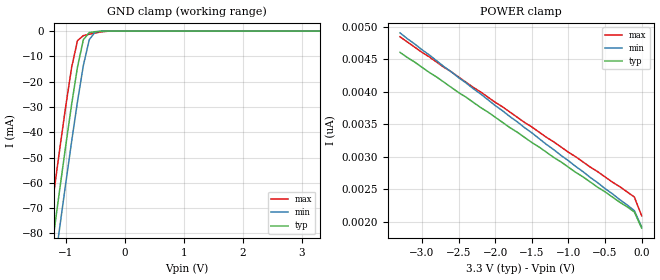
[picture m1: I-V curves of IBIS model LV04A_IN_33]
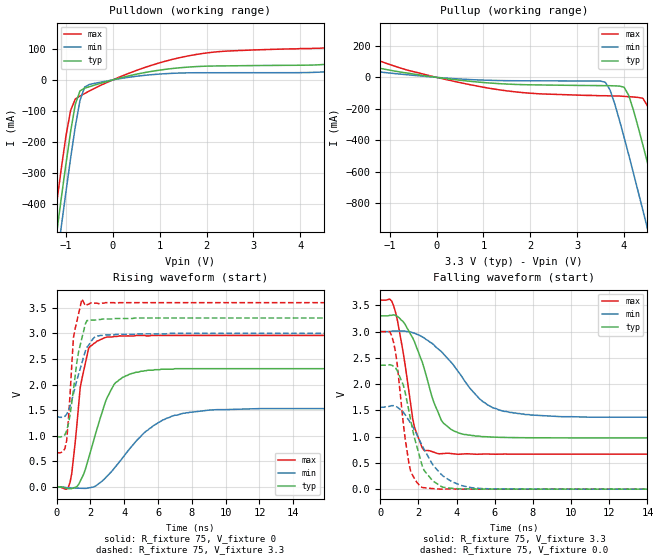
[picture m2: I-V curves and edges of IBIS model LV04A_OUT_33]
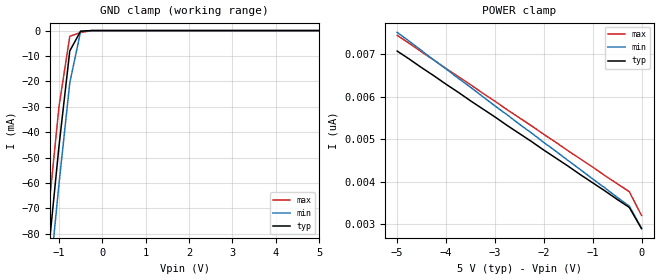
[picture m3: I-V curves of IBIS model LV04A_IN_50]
| TEXAS INSTRUMENTS INCORPORATED
| Standard Linear and Logic Group
| IBIS Model of SN74LV04A
| HEX INVERTER
| SOIC 14-pin (D), SOP 14-pin (NS), SSOP 14-pin (DB), TSSOP 14-pin (PW)
| and TVSOP 14-pin (DGV) Package
[IBIS Ver]   3.2
[Comment Char]  |_char
[File Name]   lv04a.ibs
[File Rev]   2.0 H_die
[Date]   May 26, 2000
[Source]   Data created from HSPICE simulations at TI-SLL.
[Notes]   The following is an IBIS list for the LV04A.
|   Please contact sllibis@ti.com with questions and
|   comments concerning SLL IBIS models.
|   The warning about AC Rising Endpoint might be reported,
|   but it is due to HSPICE issue and negligible.
[Disclaimer] Property of Texas Instruments Incorporated.  Unauthorized
   reproduction and/or distribution is strictly prohibited.
   This product is protected under copyright law.
   Created 2000, (C) Copyright 2000, Texas Instruments Inc.,
   All Rights Reserved.
   UNLESS THERE IS A SIGNED, WRITTEN AGREEMENT TO THE
   CONTRARY, TEXAS INSTRUMENTS () IS PROVIDING THE IBIS
   MODELS  AND WITHOUT ANY WARRANTY, EXPRESSED OR
   IMPLIED.  TI assumes no liability for:
   1) the accuracy of the IBIS models provided to your
   company;
   2) the proper functioning of these IBIS Models in your
   design or for any resulting applications; or
   3) infringement of patents, copyrights or intellectual
   property rights resulting from your use of these IBIS
   models.
   TI provides IBIS Models as a service to our customers.
   You and your company shall not distribute, sell or give
   these models to anyone else without prior written
   permission from TI.
   TI reserves the right to make changes to our products or
   to discontinue any semiconductor product or service
   without notice, and advises our customers to obtain the
   latest version of relevant information to verify, before
   placing orders, that the information being relied on is
   current.
   Please be aware that your receipt and use of the IBIS
   information provided shall serve as acceptance of these
   terms and conditions.  If you do not accept these terms,
   you should return or destroy the IBIS models and any
   other accompanying information immediately.
|   Component LV04A_D
[Component]   LV04A_D
[Manufacturer]  Texas Instruments, Inc.
[Package]
|   typ   min   max
R_pkg   0.031   0.028   0.034
L_pkg   3.109nH   2.462nH   3.889nH
C_pkg   0.473pF   0.363pF   0.628pF
[Pin]   signal_name   model_name   R_pin   L_pin   C_pin
1   1A   LV04A_IN   0.033   3.854nH   0.622pF
2   1Y   LV04A_OUT   0.032   3.188nH   0.473pF
3   2A   LV04A_IN   0.028   2.462nH   0.377pF
4   2Y   LV04A_OUT   0.031   2.596nH   0.363pF
5   3A   LV04A_IN   0.028   2.521nH   0.372pF
6   3Y   LV04A_OUT   0.034   3.250nH   0.476pF
7   GND   GND   0.034   3.889nH   0.628pF
8   4Y   LV04A_OUT   0.034   3.889nH   0.628pF
9   4A   LV04A_IN   0.034   3.250nH   0.476pF
10   5Y   LV04A_OUT   0.028   2.521nH   0.372pF
11   5A   LV04A_IN   0.031   2.596nH   0.364pF
12   6Y   LV04A_OUT   0.028   2.462nH   0.377pF
13   6A   LV04A_IN   0.032   3.188nH   0.473pF
14   VCC   POWER   0.033   3.854nH   0.622pF
|   Component LV04A_NS
[Component]   LV04A_NS
[Manufacturer]  Texas Instruments, Inc
[Package]
|   typ   min   max
R_pkg   0.045   0.039   0.054
L_pkg   3.796nH   2.561nH   4.952nH
C_pkg   0.528pF   0.288pF   0.710pF
[Pin]   signal_name   model_name   R_pin   L_pin   C_pin
1   1A   LV04A_IN   0.047   4.867nH   0.706pF
2   1Y   LV04A_OUT   0.051   4.083nH   0.592pF
3   2A   LV04A_IN   0.041   2.915nH   0.376pF
4   2Y   LV04A_OUT   0.039   2.561nH   0.288pF
5   3A   LV04A_IN   0.041   3.101nH   0.430pF
6   3Y   LV04A_OUT   0.047   4.047nH   0.589pF
7   GND   GND   0.051   4.909nH   0.700pF
8   4Y   LV04A_OUT   0.045   4.784nH   0.694pF
9   4A   LV04A_IN   0.054   4.176nH   0.597pF
10   5Y   LV04A_OUT   0.039   3.287nH   0.449pF
11   5A   LV04A_IN   0.039   2.586nH   0.294pF
12   6Y   LV04A_OUT   0.040   2.802nH   0.371pF
13   6A   LV04A_IN   0.049   4.080nH   0.593pF
14   VCC   POWER   0.052   4.952nH   0.710pF
|   Component LV04A_DB
[Component]   LV04A_DB
[Manufacturer]  Texas Instruments, Inc.
[Package]
|   typ   min   max
R_pkg   0.044   0.041   0.046
L_pkg   3.551nH   3.258nH   3.927nH
C_pkg   0.402pF   0.360pF   0.421pF
[Pin]   signal_name   model_name   R_pin   L_pin   C_pin
1   1A   LV04A_IN   0.046   3.927nH   0.408pF
2   1Y   LV04A_OUT   0.044   3.587nH   0.421pF
3   2A   LV04A_IN   0.041   3.289nH   0.398pF
4   2Y   LV04A_OUT   0.042   3.258nH   0.360pF
5   3A   LV04A_IN   0.041   3.286nH   0.403pF
6   3Y   LV04A_OUT   0.044   3.586nH   0.421pF
7   GND   GND   0.046   3.927nH   0.408pF
8   4Y   LV04A_OUT   0.046   3.927nH   0.408pF
9   4A   LV04A_IN   0.044   3.586nH   0.421pF
10   5Y   LV04A_OUT   0.041   3.286nH   0.403pF
11   5A   LV04A_IN   0.043   3.258nH   0.360pF
12   6Y   LV04A_OUT   0.041   3.289nH   0.398pF
13   6A   LV04A_IN   0.044   3.587nH   0.421pF
14   VCC   POWER   0.046   3.927nH   0.408pF
|   Component LV04A_PW
[Component]   LV04A_PW
[Manufacturer]  Texas Instruments, Inc.
[Package]
|   typ   min   max
R_pkg   0.032   0.029   0.035
L_pkg   2.378nH   2.170nH   2.680nH
C_pkg   0.314pF   0.270pF   0.335pF
[Pin]   signal_name   model_name   R_pin   L_pin   C_pin
1   1A   LV04A_IN   0.033   2.618nH   0.330pF
2   1Y   LV04A_OUT   0.031   2.313nH   0.317pF
3   2A   LV04A_IN   0.030   2.310nH   0.314pF
4   2Y   LV04A_OUT   0.031   2.173nH   0.272pF
5   3A   LV04A_IN   0.030   2.204nH   0.309pF
6   3Y   LV04A_OUT   0.032   2.315nH   0.317pF
7   GND   GND   0.035   2.680nH   0.335pF
8   4Y   LV04A_OUT   0.033   2.640nH   0.333pF
9   4A   LV04A_IN   0.034   2.347nH   0.319pF
10   5Y   LV04A_OUT   0.029   2.277nH   0.313pF
11   5A   LV04A_IN   0.031   2.170nH   0.270pF
12   6Y   LV04A_OUT   0.031   2.244nH   0.311pF
13   6A   LV04A_IN   0.033   2.343nH   0.321pF
14   VCC   POWER   0.035   2.657nH   0.332pF
|   Component LV04A_DGV
[Component]   LV04A_DGV
[Manufacturer]  Texas Instruments, Inc.
[Package]
|   typ   min   max
R_pkg   0.035   0.020   0.045
L_pkg   2.499nH   2.077nH   2.966nH
C_pkg   0.361pF   0.305pF   0.416pF
[Pin]   signal_name   model_name   R_pin   L_pin   C_pin
1   1A   LV04A_IN   0.027   2.717nH   0.373pF
2   1Y   LV04A_OUT   0.037   2.434nH   0.398pF
3   2A   LV04A_IN   0.034   2.200nH   0.316pF
4   2Y   LV04A_OUT   0.020   2.077nH   0.309pF
5   3A   LV04A_IN   0.030   2.147nH   0.305pF
6   3Y   LV04A_OUT   0.042   2.580nH   0.408pF
7   GND   GND   0.039   2.921nH   0.385pF
8   4Y   LV04A_OUT   0.033   2.841nH   0.380pF
9   4A   LV04A_IN   0.042   2.611nH   0.410pF
10   5Y   LV04A_OUT   0.038   2.331nH   0.329pF
11   5A   LV04A_IN   0.026   2.223nH   0.319pF
12   6Y   LV04A_OUT   0.034   2.259nH   0.313pF
13   6A   LV04A_IN   0.045   2.681nH   0.416pF
14   VCC   POWER   0.042   2.966nH   0.386pF
[Model Selector]   LV04A_IN
LV04A_IN_33   3.3-V Vcc Input Model
LV04A_IN_50   5.0-V Vcc Input Model
[Model Selector]   LV04A_OUT
LV04A_OUT_33   3.3-V Vcc Output Model
LV04A_OUT_50   5.0-V Vcc Output Model
| Models and submodels in the file (4): LV04A_IN_33 (Input), LV04A_OUT_33 (Output), LV04A_IN_50 (Input), LV04A_OUT_50 (Output)
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|   Model LV04A_IN_33
[Model]   LV04A_IN_33
Model_type  Input
Polarity   Inverting
Vinl = 0.99
Vinh = 2.31
| variable   typ   min   max
C_comp   1.24pf   0.94pf   1.54pf
[Temperature Range]   25   85   -40
[Voltage Range]   3.3   3.0   3.6
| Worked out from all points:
|   GND clamp passes 1 mA (typ) near -0.61 V on its own axis
[GND Clamp]
|   Voltage   I(typ)   I(min)   I(max)
-3.3V     -460mA     -475mA     -445mA
-1.3V     -97.5mA    -113mA     -81.5mA
-1.2V     -79.9mA    -95mA      -63.9mA
-1.1V     -62.6mA    -77.6mA    -46.7mA
-1V       -45.6mA    -60.5mA    -30mA
-900mV    -29.2mA    -43.9mA    -14.6mA
-800mV    -14.3mA    -28mA      -3.81mA
-700mV    -3.42mA    -13.6mA    -1.78mA
-600mV    -581uA     -3.4mA     -1.25mA
-500mV    -233uA     -353uA     -759uA
-400mV    -58.1uA    -21.9uA    -324uA
3.3V      1.9nA      2.34nA     1.69nA
[POWER Clamp]
|   Voltage   I(typ)   I(min)   I(max)
-3.3V     4.61nA     4.91nA     4.85nA
-3V       4.38nA     4.65nA     4.61nA
-100mV    2.15nA     2.17nA     2.38nA
0V        1.9nA      1.92nA     2.09nA
|   Model LV04A_OUT_33
[Model]   LV04A_OUT_33
Model_type  Output
Polarity   Non-Inverting
Vmeas = 1.65v
Cref = 15pf
| variable   typ   min   max
C_comp   4.62pf   3.47pf   5.77pf
[Temperature Range]   25   85   -40
[Voltage Range]   3.3   3.0   3.6
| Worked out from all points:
|   slope of the pulldown table from 0 to 0.495 V, typ, clamps not added: 27.3 ohm
|   slope of the pullup table from 0 to 0.495 V, typ, clamps not added: 27.2 ohm
|   rising waveform, R_fixture 75, V_fixture 0: 20-80 % time 1.34ns typ, 2.6ns min, 661ps max; typ from 0 V to 2.31 V
|   falling waveform, R_fixture 75, V_fixture 3.3: 20-80 % time 1.3ns typ, 2.26ns min, 753ps max; typ from 3.3 V to 0.976 V
|   rising waveform, R_fixture 75, V_fixture 3.3: 20-80 % time 633ps typ, 825ps min, 367ps max; typ from 0.976 V to 3.3 V
|   falling waveform, R_fixture 75, V_fixture 0.0: 20-80 % time 904ps typ, 1.52ns min, 577ps max; typ from 2.36 V to 0 V
[Pulldown]
|   Voltage   I(typ)   I(min)   I(max)
-3.3V     -3.04A     -3.13A     -2.95A
-1.3V     -615mA     -707mA     -518mA
-1.2V     -498mA     -591mA     -401mA
-1.1V     -383mA     -475mA     -288mA
-900mV    -167mA     -253mA     -98.6mA
-800mV    -79.1mA    -151mA     -61.7mA
-700mV    -35.5mA    -66.4mA    -51.9mA
-600mV    -26.8mA    -23.2mA    -43.9mA
-500mV    -22mA      -14.7mA    -35.8mA
1.6V      41.2mA     22.8mA     77.1mA
4.7V      52.1mA     27.5mA     106mA
6.6V      86.8mA     47.3mA     166mA
[Pullup]
|   Voltage   I(typ)   I(min)   I(max)
-3.3V     166mA      91.1mA     311mA
600mV     -21.6mA    -12.3mA    -39.7mA
3.6V      -52.9mA    -31.5mA    -117mA
3.8V      -54.2mA    -168mA     -119mA
4V        -62.6mA    -381mA     -121mA
4.1V      -115mA     -494mA     -123mA
4.4V      -429mA     -845mA     -133mA
4.5V      -544mA     -964mA     -182mA
4.8V      -899mA     -1.32A     -505mA
4.9V      -1.02A     -1.44A     -622mA
5.2V      -1.38A     -1.81A     -981mA
6.6V      -3.09A     -3.52A     -2.69A
[Ramp]
| variable   typ   min   max
dV/dt_r   1.40E+00/1.34E-09   9.37E-01/2.69E-09   1.78E+00/5.85E-10
dV/dt_f   1.41E+00/1.27E-09   9.88E-01/2.28E-09   1.77E+00/7.57E-10
R_load = 75
[Rising Waveform]
R_fixture = 75
V_fixture = 0
|   Time   V(typ)   V(min)   V(max)
0s        0V         0V         0V
800ps     -36.6mV    -20.1mV    88.9mV
1.1ns     -8.09mV    -23.5mV    856mV
1.4ns     111mV      -26.4mV    1.94V
1.9ns     565mV      -20mV      2.71V
2.8ns     1.57V      144mV      2.91V
3.9ns     2.14V      565mV      2.95V
5.7ns     2.28V      1.19V      2.96V
7.5ns     2.31V      1.44V      2.96V
25ns      2.31V      1.53V      2.96V
[Falling Waveform]
R_fixture = 75
V_fixture = 3.3
V_fixture_min = 3.0
V_fixture_max = 3.6
|   Time   V(typ)   V(min)   V(max)
0s        3.3V       3V         3.6V
500ps     3.31V      3V         3.62V
800ps     3.31V      3.01V      3.37V
1.7ns     2.88V      2.98V      1.34V
2.3ns     2.3V       2.88V      736mV
3.2ns     1.31V      2.62V      676mV
4.4ns     1.04V      2.07V      671mV
5.6ns     997mV      1.61V      669mV
7.6ns     979mV      1.42V      667mV
25ns      976mV      1.37V      666mV
[Rising Waveform]
R_fixture = 75
V_fixture = 3.3
V_fixture_min = 3.0
V_fixture_max = 3.6
|   Time   V(typ)   V(min)   V(max)
0s        976mV      1.37V      666mV
400ps     987mV      1.36V      696mV
600ps     1.1V       1.42V      907mV
700ps     1.23V      1.49V      1.3V
1ns       1.9V       1.82V      2.92V
1.2ns     2.43V      2.08V      3.23V
1.5ns     2.91V      2.42V      3.67V
1.8ns     3.25V      2.73V      3.56V
2.8ns     3.28V      2.97V      3.59V
25ns      3.3V       3V         3.6V
[Falling Waveform]
R_fixture = 75
V_fixture = 0.0
|   Time   V(typ)   V(min)   V(max)
0s        2.36V      1.56V      3V
500ps     2.37V      1.58V      3V
700ps     2.34V      1.59V      2.79V
900ps     2.25V      1.56V      2.34V
1.2ns     1.99V      1.47V      1.27V
1.5ns     1.49V      1.31V      490mV
2.2ns     442mV      824mV      31.6mV
3.3ns     35.3mV     247mV      1.35mV
4.8ns     4.49mV     27.2mV     1.6mV
25ns      11.4uV     564nV      13.9uV
|   Model LV04A_IN_50
[Model]   LV04A_IN_50
Model_type  Input
Polarity   Inverting
Vinl = 1.5
Vinh = 3.5
| variable   typ   min   max
C_comp   1.24pf   0.94pf   1.54pf
[Temperature Range]   25   85   -40
[Voltage Range]   5.0   4.5   5.5
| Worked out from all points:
|   GND clamp passes 1 mA (typ) near -0.52 V on its own axis
[GND Clamp]
|   Voltage   I(typ)   I(min)   I(max)
-5V       -773mA     -786mA     -758mA
-1.5V     -133mA     -148mA     -117mA
-1.25V    -88.7mA    -104mA     -72.7mA
-1V       -45.6mA    -60.5mA    -30mA
-750mV    -7.99mA    -20.5mA    -2.23mA
-500mV    -233uA     -353uA     -759uA
-250mV    -2.63nA    -182nA     -26.9uA
5V        2.9nA      3.64nA     2.54nA
[POWER Clamp]
|   Voltage   I(typ)   I(min)   I(max)
-5V       7.08nA     7.52nA     7.45nA
-1.5V     4.37nA     4.5nA      4.73nA
-250mV    3.4nA      3.43nA     3.77nA
0V        2.9nA      2.91nA     3.21nA
